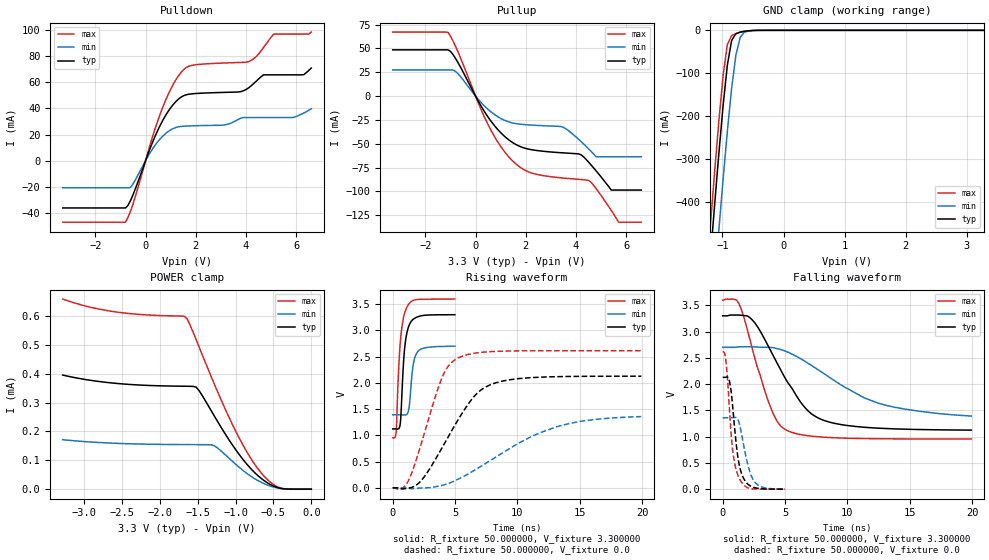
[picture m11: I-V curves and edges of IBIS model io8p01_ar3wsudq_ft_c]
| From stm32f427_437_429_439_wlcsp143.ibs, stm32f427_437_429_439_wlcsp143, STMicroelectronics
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|   Model io8p01_ar3wsudq_ft_c
[Model]  io8p01_ar3wsudq_ft_c
Model_type I/O
Polarity   Non-Inverting
Enable   Active-Low
Vinl =   0.990000V
Vinh =   2.310000V
Vmeas =  1.650000V
Cref =   50.000000pF
Rref =   100.000000M
Vref =   0.0V
C_comp   5.986400pF   5.818600pF   6.191500pF
[Temperature Range]   25.000000   0.125000k   -40.000000
[Pullup Reference]   3.300000V   2.700000V   3.600000V
[Pulldown Reference]   0.0V   0.0V   0.0V
[POWER Clamp Reference]   3.300000V   2.700000V   3.600000V
[GND Clamp Reference]   0.0V   0.0V   0.0V
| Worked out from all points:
|   slope of the pulldown table from 0 to 0.495 V, typ, clamps not added: 20.9 ohm
|   slope of the pullup table from 0 to 0.495 V, typ, clamps not added: 22.6 ohm
|   GND clamp passes 1 mA (typ) near -0.57 V on its own axis
|   rising waveform, R_fixture 50.000000, V_fixture 3.300000: 20-80 % time 372ps typ, 353ps min, 395ps max; typ from 1.12 V to 3.3 V
|   rising waveform, R_fixture 50.000000, V_fixture 0.0: 20-80 % time 3.26ns typ, 6.14ns min, 2.07ns max; typ from 0 V to 2.13 V
|   falling waveform, R_fixture 50.000000, V_fixture 3.300000: 20-80 % time 3.23ns typ, 5.72ns min, 2.03ns max; typ from 3.3 V to 1.12 V
|   falling waveform, R_fixture 50.000000, V_fixture 0.0: 20-80 % time 612ps typ, 781ps min, 546ps max; typ from 2.13 V to 0 V
[Pulldown]
|Voltage   I(typ)   I(min)   I(max)
-3.3V     -36.18mA   -20.77mA   -47.07mA
-800mV    -36.18mA   -20.77mA   -47.07mA
-600mV    -30.5mA    -20.52mA   -38.69mA
700mV     31.4mA     19.11mA    41.71mA
1.2V      45.15mA    25.37mA    61.75mA
1.6V      50.35mA    26.5mA     71.06mA
3.1V      52.28mA    27.26mA    74.75mA
4.1V      55.71mA    33.01mA    75.8mA
4.7V      65.73mA    33.01mA    86.69mA
5.1V      65.73mA    33.01mA    96.9mA
6.3V      65.85mA    36.5mA     96.9mA
6.6V      70.91mA    39.71mA    98.45mA
[Pullup]
|Voltage   I(typ)   I(min)   I(max)
-3.3V     48.54mA    27.45mA    67.16mA
-1.1V     48.54mA    27.45mA    66.87mA
-700mV    35.13mA    23.48mA    46.33mA
500mV     -22.07mA   -14mA      -30.03mA
1.5V      -49.1mA    -28.3mA    -68.56mA
2.2V      -56.05mA   -30.32mA   -80.35mA
3.5V      -59.53mA   -32.72mA   -85.92mA
4.5V      -69.2mA    -55.3mA    -88.43mA
4.8V      -78.4mA    -63.6mA    -97.01mA
5.4V      -98.5mA    -63.6mA    -119.8mA
5.7V      -98.5mA    -63.6mA    -132.2mA
6.6V      -98.5mA    -63.6mA    -132.2mA
[GND_clamp]
|Voltage   I(typ)   I(min)   I(max)
-3.3V     -4.641A    -4.8A      -4.589A
-1.2V     -535.6mA   -717.5mA   -459.3mA
-1.13V    -409.9mA   -591mA     -333.1mA
-1.06V    -288.9mA   -467.4mA   -212.9mA
-990mV    -176.2mA   -348mA     -105.7mA
-920mV    -81.01mA   -235.5mA   -32.96mA
-850mV    -23.66mA   -135.1mA   -12.27mA
-780mV    -7.753mA   -57.42mA   -7.762mA
-710mV    -4.185mA   -16.31mA   -4.763mA
-640mV    -2.295mA   -4.401mA   -2.439mA
-570mV    -1.048mA   -1.62mA    -953.6uA
3.28V     0A         0A         0A
[POWER_clamp]
|Voltage   I(typ)   I(min)   I(max)
-3.28V    395.3uA    171.4uA    658.7uA
-2.56V    366.2uA    158.7uA    613.4uA
-1.68V    356.7uA    154.5uA    599.4uA
-1.64V    356.6uA    154.5uA    590.8uA
-1.52V    353.6uA    154.3uA    518.3uA
-1.48V    341.1uA    154.3uA    492.3uA
-1.28V    253.6uA    150.4uA    364.2uA
-960mV    123.1uA    77.62uA    181.6uA
-720mV    50.52uA    32.09uA    76.18uA
-560mV    18.94uA    12.32uA    28.65uA
-440mV    5.105uA    3.74uA     7.327uA
0V        0A         0A         0A
[Ramp]
| variable   typ   min   max
dV/dt_r  1.27746/3.25923n   0.79710/6.10042n   1.56726/2.07051n
dV/dt_f  1.30206/3.22747n   0.73836/5.64214n   1.58767/2.03111n
R_load = 50.000000
[Rising Waveform]
R_fixture= 50.000000
V_fixture= 3.300000
V_fixture_min= 2.700000
V_fixture_max= 3.600000
|time   V(typ)   V(min)   V(max)
0s        1.124V     1.392V     954.2mV
280.3ps   1.124V     1.392V     1.083V
450.5ps   1.124V     1.392V     2.128V
600.6ps   1.215V     1.392V     2.753V
870.9ps   2.405V     1.39V      3.249V
1.081ns   2.884V     1.393V     3.417V
1.311ns   3.096V     1.528V     3.509V
1.652ns   3.215V     2.354V     3.573V
1.952ns   3.255V     2.578V     3.589V
4.985ns   3.3V       2.7V       3.598V
[Rising Waveform]
R_fixture= 50.000000
V_fixture= 0.0
V_fixture_min= 0.0
V_fixture_max= 0.0
|time   V(typ)   V(min)   V(max)
0s        312.9uV    184.9uV    1.351mV
840.8ps   -19.44mV   612.1uV    5.353mV
1.281ns   -4.762mV   -7.752mV   146.3mV
2.322ns   148.6mV    -2.838mV   868.7mV
3.924ns   749.9mV    43.08mV    2.081V
5.245ns   1.297V     164.7mV    2.476V
6.887ns   1.828V     382.5mV    2.576V
8.689ns   2.029V     648.6mV    2.604V
13.13ns   2.119V     1.163V     2.614V
19.94ns   2.129V     1.359V     2.614V
[Falling Waveform]
R_fixture= 50.000000
V_fixture= 3.300000
V_fixture_min= 2.700000
V_fixture_max= 3.600000
|time   V(typ)   V(min)   V(max)
0s        3.3V       2.7V       3.598V
1.321ns   3.314V     2.709V     3.52V
2.402ns   3.214V     2.71V      2.648V
3.764ns   2.673V     2.7V       1.605V
4.404ns   2.381V     2.674V     1.278V
5.085ns   2.083V     2.621V     1.127V
6.767ns   1.509V     2.409V     1.02V
8.569ns   1.276V     2.128V     983.4mV
13.17ns   1.154V     1.592V     958.3mV
19.94ns   1.124V     1.392V     954.2mV
[Falling Waveform]
R_fixture= 50.000000
V_fixture= 0.0
V_fixture_min= 0.0
V_fixture_max= 0.0
|time   V(typ)   V(min)   V(max)
0s        2.129V     1.359V     2.614V
260.3ps   2.132V     1.359V     2.439V
410.4ps   2.129V     1.358V     2.028V
580.6ps   2.008V     1.358V     1.368V
720.7ps   1.769V     1.359V     918.2mV
870.9ps   1.385V     1.362V     614.8mV
1.311ns   480.5mV    1.264V     212.8mV
1.792ns   158.8mV    701.1mV    60.62mV
2.472ns   35.88mV    168.6mV    4.67mV
4.985ns   312.9uV    184.9uV    1.351mV
